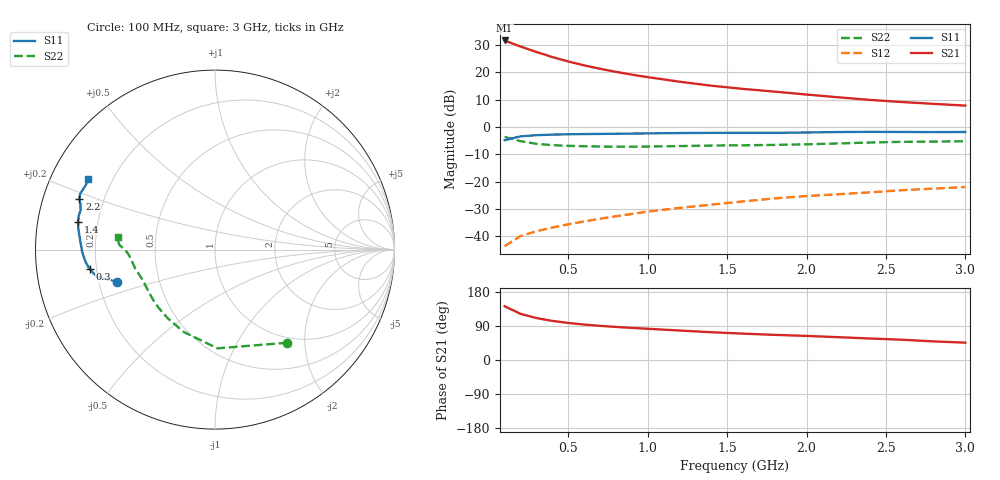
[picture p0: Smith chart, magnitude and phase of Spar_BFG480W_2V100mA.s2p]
! Filename: 2100BFG480.001
! Title: BFG480W
! Bias: Vce=2V; Ic=100mA
! Company: NXP Semiconductors NL
! User: Quality&Reliability T&D
! Measure time: 10 Nov 1999 / 11:55:01
#  MHz  S  MA  R 50
! Freq  S11  S21  S12  S22  :
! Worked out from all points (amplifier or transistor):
!   20 points, 100 MHz to 3 GHz, reference 50 ohm
!   highest |S21| = 31.6 dB at 100 MHz (marker M1)
!   |S21| within 3 dB of that: start of sweep to 239.5 MHz
!   unconditionally stable (mu >= 1): 582.6 MHz to end of sweep
!   at 400 MHz: K = 0.89, MSG = 31.1 dB, |S12| = -36.8 dB
!   at 1.2 GHz: K = 1.11, MAG = 21.0 dB, |S12| = -29.6 dB
!   at 3 GHz: K = 1.11, MAG = 12.9 dB, |S12| = -21.9 dB
!   S11 on the Smith chart (normalised r, x): 100 MHz: 0.28, -0.15; 300 MHz: 0.17, -0.08; 1.4 GHz: 0.13, +0.10; 2.2 GHz: 0.11, +0.18; 3 GHz: 0.11, +0.26
100  0.5728 -161.8  37.95 141.9  0.006639 66.7  0.657 -52.1
200  0.6723 -166.8  29.38 121.8  0.01014 58.7  0.5502 -88.5
300  0.7065 -171.1  23.43 110.7  0.01242 58.6  0.4914 -110.5
400  0.7239 -174.4  18.88 103.2  0.01452 60.4  0.4645 -124.6
500  0.7333 -177.1  15.72 97.8  0.01663 62.9  0.4515 -134.3
600  0.7411 -179.3  13.32 93.6  0.01876 64.8  0.4437 -141.2
700  0.7449 178.7  11.55 90.2  0.02106 66.8  0.4387 -146.5
800  0.7508 176.9  10.14 87.2  0.02337 68.2  0.436 -150.8
900  0.7561 175.2  9.017 84.8  0.02571 70.1  0.4358 -154.4
1000  0.7618 173.6  8.119 82.4  0.0284 70.8  0.4378 -157.7
1200  0.7725 170.7  6.701 77.8  0.03317 72.2  0.4467 -162.8
1400  0.7792 168.5  5.666 73.3  0.03804 72.8  0.4567 -166.6
1600  0.7822 166.1  4.948 69.6  0.04358 73.3  0.4622 -169.7
1800  0.7808 163.6  4.411 66.3  0.04951 73.7  0.4694 -173.0
2000  0.7905 161.4  3.904 63.6  0.05463 74.0  0.4816 -176.6
2200  0.8066 159.4  3.479 60.2  0.05891 73.9  0.4992 -179.7
2400  0.8127 157.6  3.115 56.7  0.06382 73.3  0.5195 178.4
2600  0.8094 155.8  2.849 53.5  0.06997 72.4  0.5338 177.2
2800  0.8047 153.5  2.639 49.1  0.07457 71.0  0.5399 175.3
3000  0.8085 150.8  2.451 45.8  0.07994 70.1  0.5468 172.6
